FUNCTION_BLOCK Example04_waituntil //2x1 flyways w/ 2 xbots - waituntil cmdlb,waituntil displacement
VAR_INPUT
	Execute : BOOL;
END_VAR
VAR_OUTPUT
	Done : BOOL;
END_VAR
VAR_IN_OUT
	PM_Controller : PMControllerType;	// the planar motor controller to use
END_VAR
VAR
	xbotID_array78 : ARRAY[0..77] OF USINT;
	PosX_array78 : ARRAY[0..77] OF REAL;
	PosY_array78 : ARRAY[0..77] OF REAL;
	PMC_AutoDrivingMotion1 : PMC_AutoDrivingMotion;
	PMC_XYMotion1 : PMC_XYMotion;
	PMC_WaitUntilCmdLb1 : PMC_WaitUntilCmdLb;
	PMC_XYMotion2 : PMC_XYMotion;
	Delay1 : Delay;
	PMC_XYMotion3 : PMC_XYMotion;
	PMC_WaitUntilDisp1 : PMC_WaitUntilDisp;
	PMC_XYMotion4 : PMC_XYMotion;
	PMC_XYMotion5 : PMC_XYMotion;
	PMC_WaitUntilDisp2 : PMC_WaitUntilDisp;
	PMC_XYMotion6 : PMC_XYMotion;
	PMC_XYMotion7 : PMC_XYMotion;
END_VAR

//2x1 flyways w/ 2 xbots - waituntil cmdlb,waituntil displacement

//async move to 60,60 and 60,180
xbotID_array78[0] := 1;xbotID_array78[1] := 2;
PosX_array78[0] := 0.06;PosX_array78[1] := 0.18;
PosY_array78[0] := 0.06;PosY_array78[1] := 0.06;
PMC_AutoDrivingMotion1(Execute := Execute,nXbots := 2,RoutingType := 0,ZoneID := 0,XbotID := xbotID_array78,PosX := PosX_array78,PosY := PosY_array78,PM_Controller := PM_Controller);

// xbot 2 linear move to 180,180
PMC_XYMotion1(Execute := PMC_AutoDrivingMotion1.Done,cmdLB := 2,XbotID := 2,Mode := 0,Type_ := 0,PosX := 0.18,PosY := 0.18,EndVel := 0,MaxVel := 1,MaxAcc := 10,PM_Controller := PM_Controller);

//xbot 1 wait until xbot 2 does command label 5
PMC_WaitUntilCmdLb1(Execute := PMC_XYMotion1.Done,cmdLB := 3,XbotID := 1,TriggerXID := 2,TriggerType := 0,TriggerCmdLb := 5,LabelType := 0,PM_Controller := PM_Controller);

// load command to move xbot 1 to 180,60
PMC_XYMotion2(Execute := PMC_WaitUntilCmdLb1.Ack,cmdLB := 4,XbotID := 1,Mode := 0,Type_ := 0,PosX := 0.18,PosY := 0.06,EndVel := 0,MaxVel := 1,MaxAcc := 10,PM_Controller := PM_Controller);

// delay for 1 second
Delay1(Execute := PMC_XYMotion2.Ack,Cycles := 1000);

//xbot 2 move to 300,180 w/ cmd lb 5
PMC_XYMotion3(Execute := Delay1.Done,cmdLB := 5,XbotID := 2,Mode := 0,Type_ := 0,PosX := 0.3,PosY := 0.18,EndVel := 0,MaxVel := 1,MaxAcc := 10,PM_Controller := PM_Controller);

//xbot 1 waituntil xbot 2 is x > 299.9
PMC_WaitUntilDisp1(Execute := PMC_XYMotion2.Done,cmdLB := 6,XbotID := 1,TriggerXID := 2,dispMode := 0,dispType := 0,Threshold := 0.2999,posXFactor := 0,posYFactor := 0,PM_Controller := PM_Controller);

// load command to move xbot 1 to 180,180
PMC_XYMotion4(Execute := PMC_WaitUntilDisp1.Ack,cmdLB := 7,XbotID := 1,Mode := 0,Type_ := 0,PosX := 0.18,PosY := 0.18,EndVel := 0,MaxVel := 1,MaxAcc := 10,PM_Controller := PM_Controller);

// xbot 2 to 300,60
PMC_XYMotion5(Execute := PMC_XYMotion4.Ack,cmdLB := 8,XbotID := 2,Mode := 0,Type_ := 0,PosX := 0.3,PosY := 0.06,EndVel := 0,MaxVel := 1,MaxAcc := 10,PM_Controller := PM_Controller);

// xbot 1 waituntil xbot 2 is y < 60.1 mm
PMC_WaitUntilDisp2(Execute := PMC_XYMotion4.Done,cmdLB := 9,XbotID := 1,TriggerXID := 2,dispMode := 1,dispType := 1,Threshold := 0.0601,posXFactor := 0,posYFactor := 0,PM_Controller := PM_Controller);

// load command to move xbot 1 to 420,180
PMC_XYMotion6(Execute := PMC_WaitUntilDisp2.Ack,cmdLB := 10,XbotID := 1,Mode := 0,Type_ := 0,PosX := 0.42,PosY := 0.18,EndVel := 0,MaxVel := 1,MaxAcc := 10,PM_Controller := PM_Controller);

// move xbot 2 to 420,60
PMC_XYMotion7(Execute := PMC_XYMotion6.Ack,cmdLB := 11,XbotID := 2,Mode := 0,Type_ := 0,PosX := 0.42,PosY := 0.06,EndVel := 0,MaxVel := 1,MaxAcc := 10,PM_Controller := PM_Controller);

Done := PMC_XYMotion6.Done;

END_FUNCTION_BLOCK
